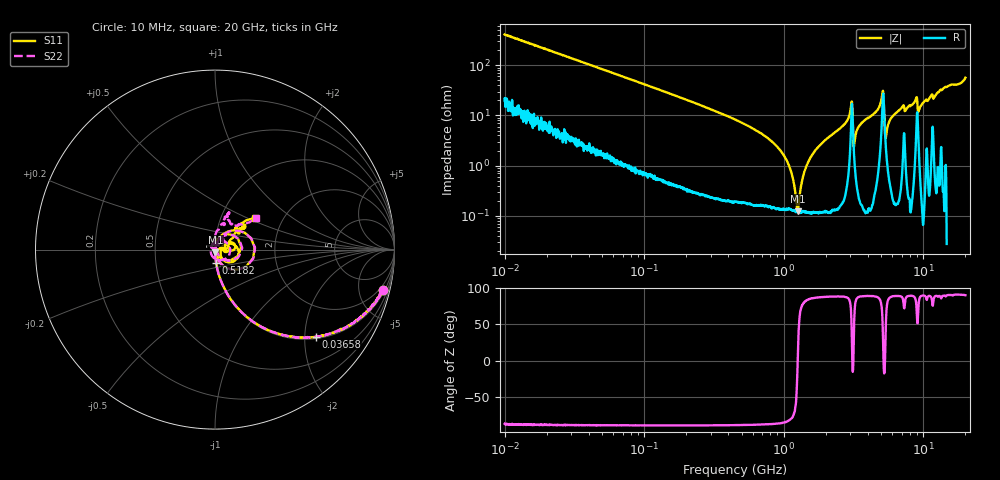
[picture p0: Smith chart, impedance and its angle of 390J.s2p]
!Keysight Technologies,P5008B,MY61100088,A.16.20.02
!Date: Tuesday, November 07, 2023 16:19:44
!Correction: S11(C  2-Port  )
!S21(C  2-Port  )
!S12(C  2-Port  )
!S22(C  2-Port  )
!S2P File: Measurements: S11, S21, S12, S22:Log Frequency Sweep
# Hz S  dB  R 50
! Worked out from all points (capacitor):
!   1601 points, 10 MHz to 20 GHz, reference 50 ohm
!   read as one part in series: C = 38.6 pF near 10.39 MHz
!   lowest |Z| = 124 mohm at 1.26 GHz (marker M1)
!   series resonance near 1.258 GHz, so ESL is about 410 pH
!   S11 on the Smith chart (normalised r, x): 10 MHz: 1.42, -8.20; 36.58 MHz: 1.05, -2.27; 518.2 MHz: 1.00, -0.15; 20 GHz: 1.45, +0.56
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1e7  -0.35 -13.5  -12.63 73.5  -12.63 73.5  -0.35 -13.5
3.555162e7  -2.48 -40.0  -3.84 48.7  -3.84 48.7  -2.48 -40.0
3.657954e7  -2.59 -40.8  -3.70 47.8  -3.70 47.8  -2.59 -40.8
1.263918e8  -10.07 -70.9  -0.49 18.1  -0.50 18.1  -10.07 -71.0
4.472136e8  -21.04 -84.2  -0.05 4.4  -0.05 4.4  -21.04 -84.4
5.181702e8  -22.51 -85.0  -0.04 3.5  -0.04 3.5  -22.51 -85.2
1.259738e9  -36.16 -79.9  -0.01 -0.9  -0.01 -0.9  -36.20 -92.5
1.589917e9  -45.81 -48.0  -0.01 -2.1  -0.01 -2.1  -47.70 -106.2
1.756711e9  -47.52 9.3  -0.01 -2.6  -0.01 -2.6  -56.63 160.8
3.033625e9  -19.14 51.0  -0.54 -10.3  -0.54 -10.3  -18.97 47.4
3.351876e9  -43.39 83.9  -0.03 -5.6  -0.03 -5.6  -40.34 29.8
3.651107e9  -32.71 89.6  -0.01 -7.1  -0.01 -7.1  -32.84 65.6
5.091486e9  -14.42 29.7  -1.30 -17.0  -1.31 -17.0  -14.31 28.5
5.652411e9  -32.32 -64.7  -0.03 -9.3  -0.04 -9.3  -35.07 -94.9
5.983999e9  -36.49 -20.1  -0.00 -11.0  -0.00 -11.0  -44.59 168.1
6.966459e9  -26.88 24.6  -0.02 -14.6  -0.02 -14.6  -28.92 108.4
8.344716e9  -27.93 16.3  0.01 -18.0  0.00 -17.9  -30.03 115.7
8.961046e9  -18.22 6.7  -0.71 -21.4  -0.71 -21.3  -21.90 21.3
9.761022e9  -29.51 -19.6  0.02 -19.7  0.01 -19.6  -32.83 163.7
1.038284e10  -26.19 12.1  -0.03 -22.3  -0.03 -22.2  -29.69 104.3
1.367661e10  -15.51 40.2  -0.10 -29.5  -0.11 -29.4  -15.69 73.5
2e10  -10.85 38.4  -0.40 -52.6  -0.40 -52.5  -10.78 37.7
